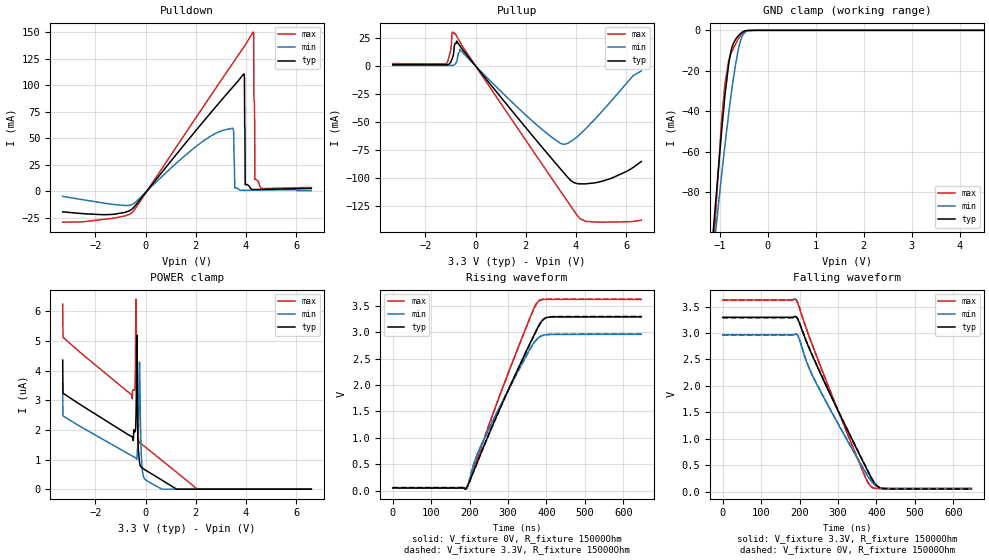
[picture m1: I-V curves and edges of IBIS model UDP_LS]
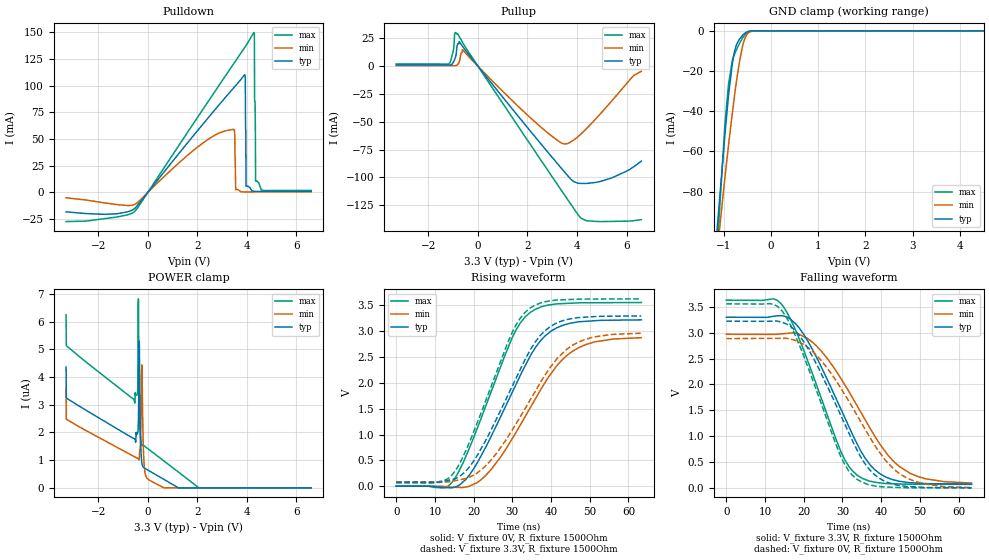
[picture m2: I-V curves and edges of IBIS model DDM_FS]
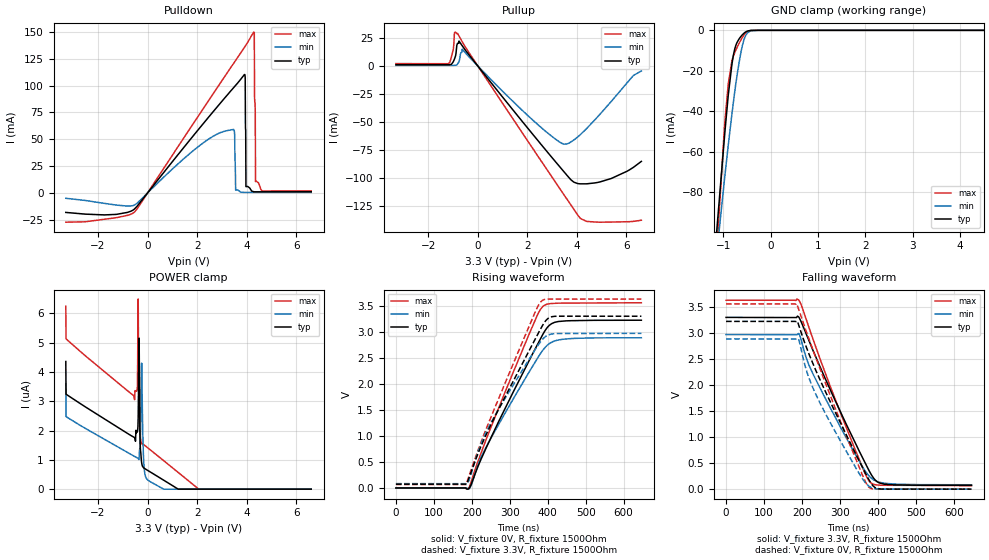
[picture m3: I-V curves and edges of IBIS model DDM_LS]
|Texas Instruments Incorporated
| ISOUSB111 Full/Low Speed Isolated USB Repeater
| Marketing Part # : ISOUSB111
| Package-type: SOIC
| #pins/pkg drawing : 16-pin DW
[IBIS Ver] 4.1
[File name] isousb111.ibs
[File Rev] 1.0
[Date] 07/25/2022
[Source]
| Texas Instruments Incorporated.
| 12500 TI Blvd
| Dallas, TX -75243
[Notes] Revision History:
| Rev 1.0: 05/25/2022
| - Initial version of the model
| - Model generated from simulations in TISPICE/SPECTRE
| - C_comp although listed in numerical order of value are
| obtained from varying PVT conditions. For PVT conditions for
| each specific value refer the buffer description under
| respective [Model]. IBIS model user is responsible for using
| appropriate C_comp to simulate for Signal Integrity.
| - Warnings regarding combined Non-monotonicity of various models have been
| reviewed and considered minor and can be ignored.
[Disclaimer]
| This model is designed as an aid for customers of Texas Instruments.
| TI and its licensors and suppliers make no warranties, either expressed
| or implied, with respect to this model, including the warranties of
| merchantability or fitness for a particular purpose. The model is
| provided solely on an "as is" basis. The entire risk as to its quality
| and performance is with the customer.
| This model is subject to change without notice. Texas Instruments
| Incorporated is not responsible for updating this model.
[Copyright]
(C) Copyright 2022 Texas Instruments Incorporated. All rights reserved.
[Component] ISOUSB111
[Manufacturer] Texas Instruments Incorporated
[Package]
R_pkg 0.05 0.04 0.06
L_pkg 1.5nH 1.2nH 2nH
C_pkg 0.2pF 0.16pF 0.24pF
| pin number (pin name) mapping to model name
[Pin] signal_name  model_name   R_pin   L_pin   C_pin
1   VBUS1   Power   0 0 0
2   GND1   GND   0 0 0
3   V3P3V1   Power   0 0 0
4   NC   NC   0 0 0
5   NC   NC   0 0 0
6   UDM   UDM   0 0 0
7   UDP   UDP   0 0 0
8   GND1   GND   0 0 0
9   GND2   GND   0 0 0
10   DDP   DDP   0 0 0
11   DDM   DDM   0 0 0
12   PIN   NC   0 0 0
13   NC   NC   0 0 0
14   V3P3V2   Power   0 0 0
15   GND2   GND   0 0 0
16   VBUS2   GND   0 0 0
[Model Selector]   UDP
UDP_FS   upstream_positive_full_speed_mode
UDP_LS   upstream_positive_low_speed_mode
[Model Selector]   UDM
UDM_FS   upstream_negative_full_speed_mode
UDM_LS   upstream_negative_low_speed_mode
[Model Selector]   DDP
DDP_FS   downstream_positive_full_speed_mode
DDP_LS   downstream_positive_low_speed_mode
[Model Selector]   DDM
DDM_FS   downstream_negative_full_speed_mode
DDM_LS   downstream_negative_low_speed_mode
| Models and submodels in the file (8): UDP_LS (I/O), DDM_FS (I/O), DDM_LS (I/O), DDP_FS (I/O), DDP_LS (I/O), UDM_FS (I/O), UDM_LS (I/O), UDP_FS (I/O)
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[Model]   UDP_LS
Model_type   I/O
Polarity   Non-Inverting
Enable   Active-Low
Vinl = 0.8
Vinh = 2
Vmeas = 1.65
Vref = 1.65
Cref = 7pF
Rref = 15000
|   typ   min   max
C_comp   8pF   5pF   10pF
[Voltage Range]   3.3   2.97   3.63
[Temperature Range]   27   150   -40
[Pullup Reference]   3.3   2.97   3.63
[Pulldown Reference]   -0   -0   -0
[Power Clamp Reference]   3.3   2.97   3.63
[GND Clamp Reference]   0   0   0
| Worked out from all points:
|   slope of the pulldown table from 0 to 0.495 V, typ, clamps not added: 33.7 ohm
|   slope of the pullup table from 0 to 0.495 V, typ, clamps not added: 35.8 ohm
|   GND clamp passes 1 mA (typ) near -0.54 V on its own axis
|   falling waveform, V_fixture 3.3V, R_fixture 15000Ohm: 20-80 % time 127ns typ, 128ns min, 116ns max; typ from 3.3 V to 0.057 V
|   rising waveform, V_fixture 0V, R_fixture 15000Ohm: 20-80 % time 119ns typ, 117ns min, 110ns max; typ from 0.05 V to 3.29 V
|   rising waveform, V_fixture 3.3V, R_fixture 15000Ohm: 20-80 % time 119ns typ, 118ns min, 110ns max; typ from 0.057 V to 3.3 V
|   falling waveform, V_fixture 0V, R_fixture 15000Ohm: 20-80 % time 127ns typ, 128ns min, 117ns max; typ from 3.29 V to 0.05 V
[Pulldown]
|   Voltage   I(typ)   I(min)   I(max)
-3.3V     -19.54mA   -4.929mA   -29.33mA
-537.9mV  -16.94mA   -12.7mA    -20.3mA
3.462V    97.95mA    59.28mA    120.4mA
3.511V    99.28mA    54.08mA    122.1mA
3.551V    100.4mA    2.78mA     123.5mA
3.917V    110.6mA    791.1uA    136.2mA
3.937V    107.2mA    798uA      136.9mA
3.967V    6.132mA    808.4uA    138mA
4.283V    1.558mA    916.9uA    150.1mA
4.343V    1.509mA    936.8uA    70.94mA
4.353V    1.513mA    940.1uA    10.95mA
6.6V      2.508mA    452.9uA    3.524mA
[GND Clamp]
|   Voltage   I(typ)   I(min)   I(max)
-3.3V     -1.286A    -1.121A    -1.579A
-1.3V     -145.3mA   -147.2mA   -170.6mA
-973.5mV  -52.59mA   -73.66mA   -47.68mA
-894.3mV  -32.06mA   -56.81mA   -26.49mA
-815.1mV  -16.5mA    -41.06mA   -14.88mA
-785.4mV  -12.23mA   -35.46mA   -12.65mA
-735.9mV  -7.575mA   -26.62mA   -9.853mA
-627mV    -3.033mA   -10.97mA   -4.745mA
-567.6mV  -1.539mA   -5.066mA   -2.489mA
-498.3mV  -471.8uA   -1.571mA   -746.6uA
-260.7mV  0A         -5.306uA   0A
6.6V      0A         0A         0A
[Pullup]
|   Voltage   I(typ)   I(min)   I(max)
-3.3V     1.142mA    462.8uA    2.096mA
-1.181V   1.061mA    442.2uA    1.943mA
-993.3mV  3.404mA    441.8uA    13.88mA
-933.9mV  6.371mA    532.5uA    29.69mA
-815.1mV  20.2mA     1.602mA    29.2mA
-627mV    18.13mA    15.01mA    21.78mA
2.095V    -57.8mA    -45.93mA   -69.71mA
3.531V    -96.08mA   -70.07mA   -117mA
3.877V    -104mA     -66.31mA   -128.3mA
4.382V    -105.6mA   -56.28mA   -139.1mA
5.392V    -100.7mA   -31.65mA   -139.8mA
6.6V      -85.53mA   -4.484mA   -138.2mA
[POWER Clamp]
|   Voltage   I(typ)   I(min)   I(max)
-3.3V     4.356uA    3.599uA    6.246uA
-3.29V    3.241uA    2.478uA    5.13uA
-528mV    1.759uA    1.119uA    3.051uA
-419.1mV  1.943uA    1.069uA    3.389uA
-379.5mV  2.53uA     1.044uA    6.418uA
-349.8mV  5.208uA    1.013uA    3.192uA
-310.2mV  1.899uA    1.42uA     1.946uA
-250.8mV  973.2nA    4.16uA     1.567uA
-171.6mV  741.5nA    1.215uA    1.531uA
-62.7mV   674.3nA    384.4nA    1.457uA
2.056V    0A         0A         4.459nA
6.6V      0A         0A         0A
[Ramp]
R_load = 15000
|   typ   min   max
dV/dt_r   1.94404/1.18803e-07   1.74728/1.17376e-07   2.13944/1.09801e-07
dV/dt_f   1.94431/1.26859e-07   1.74734/1.27745e-07   2.13971/1.1642e-07
[Falling Waveform]
V_fixture = 3.3V
V_fixture_min = 2.97V
V_fixture_max = 3.63V
R_fixture = 15000Ohm
C_fixture = 0F
|   Time   V(typ)   V(min)   V(max)
0s        3.298V     2.968V     3.627V
191.1ns   3.304V     2.98V      3.625V
199.7ns   3.189V     2.877V     3.472V
223.7ns   2.734V     2.351V     2.958V
248ns     2.335V     1.983V     2.49V
369.6ns   501mV      386.8mV    297.9mV
384.7ns   285.7mV    216.3mV    103.3mV
400.7ns   112.8mV    101.1mV    61.56mV
419.8ns   59.09mV    64.55mV    61.44mV
646.7ns   57.28mV    56mV       61.04mV
[Rising Waveform]
V_fixture = 0V
V_fixture_min = 0V
V_fixture_max = 0V
R_fixture = 15000Ohm
C_fixture = 0F
|   Time   V(typ)   V(min)   V(max)
0s        49.91mV    47.52mV    54.29mV
191.1ns   46.69mV    31.65mV    55.44mV
219ns     523.2mV    674.9mV    589.8mV
249.7ns   1.064V     1.165V     1.233V
341.4ns   2.547V     2.475V     2.986V
369.6ns   2.974V     2.825V     3.485V
379.6ns   3.119V     2.899V     3.591V
393.2ns   3.251V     2.945V     3.619V
411.8ns   3.289V     2.958V     3.621V
646.7ns   3.29V      2.96V      3.62V
[Rising Waveform]
V_fixture = 3.3V
V_fixture_min = 2.97V
V_fixture_max = 3.63V
R_fixture = 15000Ohm
C_fixture = 0F
|   Time   V(typ)   V(min)   V(max)
0s        57.28mV    56mV       61.04mV
192.3ns   59.23mV    43.25mV    63.05mV
219ns     518.2mV    668.7mV    587.9mV
249.7ns   1.058V     1.156V     1.232V
334.3ns   2.431V     2.369V     2.854V
365.8ns   2.911V     2.776V     3.42V
379.6ns   3.113V     2.894V     3.592V
391ns     3.235V     2.939V     3.625V
405.6ns   3.289V     2.958V     3.626V
646.7ns   3.298V     2.968V     3.627V
[Falling Waveform]
|Gnd
V_fixture = 0V
V_fixture_min = 0V
V_fixture_max = 0V
R_fixture = 15000Ohm
C_fixture = 0F
|   Time   V(typ)   V(min)   V(max)
0s        3.29V      2.96V      3.62V
191.1ns   3.308V     2.979V     3.63V
199.7ns   3.195V     2.882V     3.474V
223.7ns   2.737V     2.357V     2.96V
248ns     2.342V     1.992V     2.492V
365.8ns   564.5mV    444.8mV    366mV
384.7ns   290.9mV    224.8mV    103.8mV
400.7ns   115.6mV    105.6mV    59.55mV
419.8ns   55.91mV    62.81mV    55.52mV
646.7ns   49.91mV    47.52mV    54.29mV
[Model]   DDM_FS
Model_type   I/O
Polarity   Non-Inverting
Enable   Active-Low
Vinl = 0.8
Vinh = 2
Vmeas = 1.65
Vref = 1.65
Cref = 7pF
Rref = 15000
|   typ   min   max
C_comp   8pF   5pF   10pF
[Voltage Range]   3.3   2.97   3.63
[Temperature Range]   27   150   -40
[Pullup Reference]   3.3   2.97   3.63
[Pulldown Reference]   0   0   -0
[Power Clamp Reference]   3.3   2.97   3.63
[GND Clamp Reference]   0   0   0
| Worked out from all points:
|   slope of the pulldown table from 0 to 0.495 V, typ, clamps not added: 34.2 ohm
|   slope of the pullup table from 0 to 0.495 V, typ, clamps not added: 35.8 ohm
|   GND clamp passes 1 mA (typ) near -0.54 V on its own axis
|   falling waveform, V_fixture 3.3V, R_fixture 1500Ohm: 20-80 % time 12.3ns typ, 14.3ns min, 10.5ns max; typ from 3.3 V to 0.074 V
|   rising waveform, V_fixture 0V, R_fixture 1500Ohm: 20-80 % time 12.7ns typ, 14.1ns min, 11.1ns max; typ from 0 V to 3.22 V
|   rising waveform, V_fixture 3.3V, R_fixture 1500Ohm: 20-80 % time 12.9ns typ, 14.5ns min, 11.1ns max; typ from 0.073 V to 3.3 V
|   falling waveform, V_fixture 0V, R_fixture 1500Ohm: 20-80 % time 12.4ns typ, 14.5ns min, 10.6ns max; typ from 3.22 V to 0 V
[Pulldown]
|   Voltage   I(typ)   I(min)   I(max)
-3.3V     -18.2mA    -5.025mA   -27.3mA
-537.9mV  -15.2mA    -11.4mA    -18.05mA
3.452V    97.57mA    59.15mA    120.1mA
3.551V    100.2mA    2.565mA    123.5mA
3.917V    110.3mA    416.6uA    136mA
3.937V    106.9mA    416.6uA    136.7mA
3.967V    5.849mA    416.6uA    137.7mA
4.283V    1.079mA    416.7uA    149.8mA
4.303V    992.1uA    416.7uA    149.2mA
4.313V    991.4uA    416.7uA    86.59mA
4.353V    991.8uA    416.8uA    10.6mA
6.6V      1.045mA    452.9uA    1.865mA
[GND Clamp]
|   Voltage   I(typ)   I(min)   I(max)
-3.3V     -1.286A    -1.12A     -1.579A
-1.3V     -145.3mA   -147.2mA   -170.6mA
-973.5mV  -52.59mA   -73.66mA   -47.69mA
-894.3mV  -32.06mA   -56.82mA   -26.49mA
-815.1mV  -16.5mA    -41.06mA   -14.88mA
-785.4mV  -12.23mA   -35.46mA   -12.65mA
-735.9mV  -7.575mA   -26.62mA   -9.854mA
-627mV    -3.033mA   -10.97mA   -4.745mA
-567.6mV  -1.539mA   -5.066mA   -2.489mA
-498.3mV  -471.8uA   -1.572mA   -746.7uA
-260.7mV  0A         -5.306uA   0A
6.6V      0A         0A         0A
[Pullup]
|   Voltage   I(typ)   I(min)   I(max)
-3.3V     1.143mA    463.1uA    2.098mA
-1.181V   1.062mA    442.4uA    1.969mA
-993.3mV  3.464mA    442uA      14.04mA
-933.9mV  6.443mA    534.3uA    29.81mA
-815.1mV  20.24mA    1.625mA    29.16mA
-627mV    18.1mA     15mA       21.74mA
1.957V    -54.06mA   -43.1mA    -65.17mA
3.491V    -95.06mA   -70.03mA   -115.7mA
3.868V    -103.9mA   -66.45mA   -128mA
4.382V    -105.5mA   -56.25mA   -139.1mA
5.402V    -100.6mA   -31.33mA   -139.7mA
6.6V      -85.42mA   -4.486mA   -138.1mA
[POWER Clamp]
|   Voltage   I(typ)   I(min)   I(max)
-3.3V     4.356uA    3.599uA    6.245uA
-3.29V    3.24uA     2.477uA    5.129uA
-528mV    1.759uA    1.119uA    3.056uA
-409.2mV  1.967uA    1.064uA    3.479uA
-379.5mV  2.466uA    1.044uA    6.817uA
-349.8mV  5.299uA    1.01uA     3.356uA
-290.4mV  1.653uA    1.775uA    1.768uA
-250.8mV  990.4nA    4.213uA    1.556uA
-171.6mV  742.1nA    1.255uA    1.531uA
-62.7mV   674.2nA    386.2nA    1.457uA
2.056V    0A         0A         4.44nA
6.6V      0A         0A         0A
[Ramp]
R_load = 1500
|   typ   min   max
dV/dt_r   1.93262/1.26758e-08   1.7258/1.41041e-08   2.1342/1.10067e-08
dV/dt_f   1.93485/1.22744e-08   1.7255/1.42298e-08   2.13627/1.05125e-08
[Falling Waveform]
V_fixture = 3.3V
V_fixture_min = 2.97V
V_fixture_max = 3.63V
R_fixture = 1500Ohm
C_fixture = 0F
|   Time   V(typ)   V(min)   V(max)
0s        3.298V     2.969V     3.628V
14.55ns   3.324V     2.979V     3.522V
17.92ns   3.171V     2.984V     3.041V
22.88ns   2.584V     2.773V     2.078V
29.72ns   1.502V     2.098V     678.8mV
33.83ns   844.9mV    1.58V      243.3mV
38.29ns   354.9mV    1.008V     109.5mV
44.81ns   126.3mV    407.8mV    74.94mV
51.52ns   83.59mV    174.8mV    69.48mV
63.33ns   73.73mV    92.92mV    67.43mV
[Rising Waveform]
V_fixture = 0V
V_fixture_min = 0V
V_fixture_max = 0V
R_fixture = 1500Ohm
C_fixture = 0F
|   Time   V(typ)   V(min)   V(max)
0s        7.21nV     276nV      6.379nV
12.02ns   -25.13mV   -1.021mV   -31.53mV
14.55ns   -28.04mV   -21.32mV   87.57mV
17.92ns   127.4mV    -16.65mV   565.1mV
22.88ns   720.2mV    189.9mV    1.502V
30.16ns   1.847V     944.2mV    2.908V
34.59ns   2.517V     1.515V     3.364V
40.02ns   3.004V     2.182V     3.516V
45.64ns   3.165V     2.617V     3.546V
63.33ns   3.221V     2.876V     3.557V
[Rising Waveform]
V_fixture = 3.3V
V_fixture_min = 2.97V
V_fixture_max = 3.63V
R_fixture = 1500Ohm
C_fixture = 0F
|   Time   V(typ)   V(min)   V(max)
0s        73.38mV    83.93mV    67.42mV
10.05ns   74.06mV    82.64mV    70.96mV
15.13ns   142mV      106mV      283.6mV
18.84ns   367mV      174.1mV    839.2mV
24.36ns   1.069V     494.6mV    1.901V
30.07ns   1.952V     1.101V     2.994V
34.4ns    2.607V     1.643V     3.439V
39.75ns   3.089V     2.299V     3.589V
45.64ns   3.249V     2.733V     3.618V
63.33ns   3.298V     2.963V     3.628V
[Falling Waveform]
|Gnd
V_fixture = 0V
V_fixture_min = 0V
V_fixture_max = 0V
R_fixture = 1500Ohm
C_fixture = 0F
|   Time   V(typ)   V(min)   V(max)
0s        3.222V     2.885V     3.557V
11.28ns   3.221V     2.889V     3.561V
14.55ns   3.195V     2.89V      3.404V
18.84ns   2.946V     2.817V     2.761V
22.88ns   2.449V     2.595V     1.969V
29.64ns   1.389V     1.918V     592.2mV
33.63ns   753.5mV    1.42V      172.6mV
39.25ns   198.2mV    720mV      28.06mV
45.64ns   36.48mV    232.3mV    4.575mV
63.33ns   223.6uV    5.519mV    8.818uV
[Model]   DDM_LS
Model_type   I/O
Polarity   Non-Inverting
Enable   Active-Low
Vinl = 0.8
Vinh = 2
Vmeas = 1.65
Vref = 1.65
Cref = 7pF
Rref = 15000
|   typ   min   max
C_comp   8pF   5pF   10pF
[Voltage Range]   3.3   2.97   3.63
[Temperature Range]   27   150   -40
[Pullup Reference]   3.3   2.97   3.63
[Pulldown Reference]   -0   0   -0
[Power Clamp Reference]   3.3   2.97   3.63
[GND Clamp Reference]   0   0   0
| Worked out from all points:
|   slope of the pulldown table from 0 to 0.495 V, typ, clamps not added: 34.2 ohm
|   slope of the pullup table from 0 to 0.495 V, typ, clamps not added: 35.8 ohm
|   GND clamp passes 1 mA (typ) near -0.54 V on its own axis
|   falling waveform, V_fixture 3.3V, R_fixture 1500Ohm: 20-80 % time 122ns typ, 123ns min, 112ns max; typ from 3.3 V to 0.073 V
|   rising waveform, V_fixture 0V, R_fixture 1500Ohm: 20-80 % time 130ns typ, 134ns min, 118ns max; typ from 0 V to 3.22 V
|   rising waveform, V_fixture 3.3V, R_fixture 1500Ohm: 20-80 % time 133ns typ, 130ns min, 121ns max; typ from 0.073 V to 3.3 V
|   falling waveform, V_fixture 0V, R_fixture 1500Ohm: 20-80 % time 124ns typ, 118ns min, 114ns max; typ from 3.22 V to 0 V
[Pulldown]
|   Voltage   I(typ)   I(min)   I(max)
-3.3V     -18.2mA    -5.021mA   -27.31mA
-537.9mV  -15.2mA    -11.4mA    -18.05mA
3.462V    97.83mA    59.09mA    120.4mA
3.511V    99.15mA    54.21mA    122.1mA
3.551V    100.2mA    2.553mA    123.5mA
3.917V    110.3mA    416.7uA    136mA
3.937V    107.1mA    416.7uA    136.7mA
3.967V    5.835mA    416.7uA    137.7mA
4.283V    1.082mA    416.8uA    149.8mA
4.343V    991.9uA    416.8uA    75.26mA
4.353V    991.9uA    416.8uA    10.57mA
6.6V      1.045mA    453uA      1.865mA
[GND Clamp]
|   Voltage   I(typ)   I(min)   I(max)
-3.3V     -1.286A    -1.12A     -1.579A
-1.3V     -145.3mA   -147.2mA   -170.6mA
-973.5mV  -52.59mA   -73.66mA   -47.69mA
-894.3mV  -32.06mA   -56.82mA   -26.49mA
-815.1mV  -16.5mA    -41.06mA   -14.88mA
-785.4mV  -12.23mA   -35.46mA   -12.65mA
-735.9mV  -7.575mA   -26.62mA   -9.854mA
-627mV    -3.033mA   -10.97mA   -4.745mA
-567.6mV  -1.539mA   -5.066mA   -2.489mA
-498.3mV  -471.8uA   -1.572mA   -746.7uA
-260.7mV  0A         -5.306uA   0A
6.6V      0A         0A         0A
[Pullup]
|   Voltage   I(typ)   I(min)   I(max)
-3.3V     1.143mA    463.2uA    2.098mA
-1.181V   1.062mA    442.5uA    1.976mA
-993.3mV  3.479mA    442.1uA    14.08mA
-933.9mV  6.461mA    534.8uA    29.84mA
-815.1mV  20.25mA    1.633mA    29.15mA
-627mV    18.1mA     14.99mA    21.73mA
1.957V    -54.06mA   -43.1mA    -65.18mA
3.491V    -95.07mA   -70.04mA   -115.8mA
3.868V    -103.9mA   -66.47mA   -128mA
4.392V    -105.5mA   -56.05mA   -139.2mA
5.392V    -100.7mA   -31.61mA   -139.8mA
6.6V      -85.45mA   -4.491mA   -138.1mA
[POWER Clamp]
|   Voltage   I(typ)   I(min)   I(max)
-3.3V     4.356uA    3.599uA    6.245uA
-3.29V    3.24uA     2.477uA    5.129uA
-528mV    1.757uA    1.119uA    3.054uA
-409.2mV  1.968uA    1.064uA    3.496uA
-379.5mV  2.484uA    1.044uA    6.487uA
-349.8mV  5.156uA    1.012uA    3.244uA
-310.2mV  1.922uA    1.418uA    1.96uA
-250.8mV  977.8nA    4.148uA    1.565uA
-171.6mV  739.8nA    1.22uA     1.531uA
-62.7mV   674.2nA    384.7nA    1.457uA
2.056V    0A         0A         4.44nA
6.6V      0A         0A         0A
[Ramp]
R_load = 1500
|   typ   min   max
dV/dt_r   1.93315/1.30202e-07   1.73109/1.34063e-07   2.13437/1.18482e-07
dV/dt_f   1.93521/1.22049e-07   1.73101/1.23353e-07   2.13644/1.11725e-07
[Falling Waveform]
V_fixture = 3.3V
V_fixture_min = 2.97V
V_fixture_max = 3.63V
R_fixture = 1500Ohm
C_fixture = 0F
|   Time   V(typ)   V(min)   V(max)
0s        3.299V     2.969V     3.628V
191.3ns   3.307V     2.988V     3.634V
211.3ns   2.979V     2.523V     3.26V
229.4ns   2.659V     2.207V     2.875V
337.2ns   937.5mV    714.8mV    812.7mV
367.2ns   495.1mV    343.8mV    286.9mV
380.6ns   305mV      224.8mV    126.7mV
397.6ns   146.1mV    148.1mV    80.38mV
417.8ns   94.49mV    114.6mV    74.54mV
646.7ns   73.38mV    83.97mV    67.42mV
[Rising Waveform]
V_fixture = 0V
V_fixture_min = 0V
V_fixture_max = 0V
R_fixture = 1500Ohm
C_fixture = 0F
|   Time   V(typ)   V(min)   V(max)
0s        7.209nV    274.9nV    6.38nV
191.3ns   -16.21mV   -16.46mV   -7.616mV
199.1ns   84.02mV    64.94mV    138.4mV
224.3ns   551.5mV    589.6mV    669.9mV
249.2ns   945.7mV    940.3mV    1.144V
371.6ns   2.737V     2.475V     3.303V
391.1ns   3V         2.683V     3.508V
404.8ns   3.127V     2.775V     3.538V
427.6ns   3.197V     2.842V     3.549V
646.7ns   3.222V     2.885V     3.557V
[Rising Waveform]
V_fixture = 3.3V
V_fixture_min = 2.97V
V_fixture_max = 3.63V
R_fixture = 1500Ohm
C_fixture = 0F
|   Time   V(typ)   V(min)   V(max)
0s        73.38mV    83.94mV    67.42mV
184.2ns   73.41mV    82.37mV    63.66mV
191ns     166.5mV    121mV      198.8mV
221.9ns   762mV      806.5mV    835.8mV
251ns     1.227V     1.261V     1.371V
367.2ns   2.861V     2.66V      3.382V
386.1ns   3.119V     2.855V     3.604V
400.5ns   3.255V     2.935V     3.627V
417.8ns   3.297V     2.963V     3.628V
646.7ns   3.299V     2.969V     3.628V
[Falling Waveform]
|Gnd
V_fixture = 0V
V_fixture_min = 0V
V_fixture_max = 0V
R_fixture = 1500Ohm
C_fixture = 0F
|   Time   V(typ)   V(min)   V(max)
0s        3.222V     2.885V     3.557V
186ns     3.222V     2.883V     3.561V
191.3ns   3.154V     2.876V     3.455V
214.5ns   2.671V     2.22V      2.966V
244ns     2.159V     1.706V     2.38V
345.3ns   623.2mV    366.6mV    518.1mV
376.2ns   182.6mV    58.28mV    37.7mV
391.5ns   35.42mV    11.2mV     -521.7uV
410.5ns   865.8uV    1.756mV    -482.9uV
646.7ns   35.26nV    -1.726uV   59.6nV
